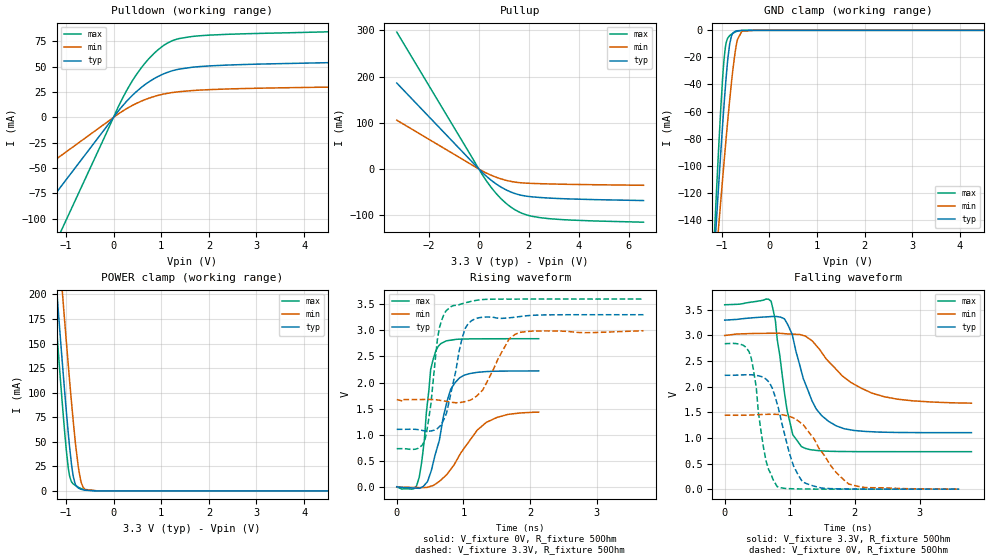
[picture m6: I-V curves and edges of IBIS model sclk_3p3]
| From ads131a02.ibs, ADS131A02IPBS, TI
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|   sclk_3p3 Model
[Model]   sclk_3p3
Model_type   I/O
Polarity   Non-Inverting
Enable   Active-Low
Vinl = 0.66
Vinh = 2.64
Vmeas = 1.65
Vref = 0
Cref = 2pF
Rref = 70
|   typ   min   max
|   (nom PVT)   (fast PVT)   (slow PVT)
C_comp   1.607e-12   1.574e-12   1.668e-12
| Where nom  PVT is Nominal Process, 3.3V, 27C
|   Fast PVT is Strong Process,  3.6V, -40C
|   Slow PVT is Weak Process,   3V, 125C
[Voltage Range]   3.3   3   3.6
|Junction Temperature
[Temperature Range]   27   125   -40
[Pullup Reference]   3.3   3   3.6
[Pulldown Reference]   0   0   0
[Power Clamp Reference]   3.3   3   3.6
[GND Clamp Reference]   0   0   0
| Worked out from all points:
|   slope of the pulldown table from 0 to 0.495 V, typ, clamps not added: 19.1 ohm
|   slope of the pullup table from 0 to 0.495 V, typ, clamps not added: 20.5 ohm
|   GND clamp passes 1 mA (typ) near -0.73 V on its own axis
|   POWER clamp passes 1 mA (typ) near -0.63 V on its own axis
|   falling waveform, V_fixture 3.3V, R_fixture 50Ohm: 20-80 % time 356ps typ, 695ps min, 204ps max; typ from 3.3 V to 1.1 V
|   rising waveform, V_fixture 0V, R_fixture 50Ohm: 20-80 % time 244ps typ, 480ps min, 130ps max; typ from 0 V to 2.22 V
|   rising waveform, V_fixture 3.3V, R_fixture 50Ohm: 20-80 % time 213ps typ, 317ps min, 156ps max; typ from 1.1 V to 3.3 V
|   falling waveform, V_fixture 0V, R_fixture 50Ohm: 20-80 % time 280ps typ, 476ps min, 184ps max; typ from 2.22 V to 0 V
[Pulldown]
|   Voltage   I(typ)   I(min)   I(max)
-3.3V     -203.7mA   -112.7mA   -335.5mA
-153.6mV  -9.48mA    -5.244mA   -15.61mA
153mV     9.485mA    5.137mA    15.86mA
462mV     24.81mA    13.45mA    41.17mA
656.7mV   32.33mA    17.49mA    53.5mA
858mV     38.51mA    20.75mA    63.65mA
1.038V    42.77mA    22.92mA    70.67mA
1.214V    45.82mA    24.42mA    75.43mA
1.647V    49.49mA    26.48mA    79.92mA
2.042V    50.92mA    27.47mA    81.33mA
5.441V    54.93mA    30.54mA    85.61mA
6.6V      57.39mA    32.04mA    89.3mA
[GND Clamp]
|   Voltage   I(typ)   I(min)   I(max)
-3.3V     -1.489A    -1.173A    -1.877A
-1.197V   -188.2mA   -201mA     -180.7mA
-1.115V   -140.9mA   -165.1mA   -120mA
-1.076V   -118.9mA   -148.3mA   -92.5mA
-985.2mV  -70.27mA   -110.1mA   -35.72mA
-924mV    -40.72mA   -85.13mA   -11.88mA
-838.2mV  -10.5mA    -52.28mA   -3.986mA
-720mV    -732.9uA   -15.72mA   -1.234mA
-672mV    -304.1uA   -6.767mA   -613.8uA
-582mV    -52.5uA    -738.4uA   -104.3uA
-330mV    -89.41nA   -746.6nA   -56.53nA
6.6V      0A         0A         0A
[Pullup]
|   Voltage   I(typ)   I(min)   I(max)
-3.3V     186.2mA    105.9mA    296.5mA
163.2mV   -8.864mA   -4.883mA   -14.59mA
462mV     -22.94mA   -12.6mA    -37.71mA
660mV     -30.98mA   -16.95mA   -50.94mA
1.15V     -46.47mA   -25.05mA   -76.84mA
1.449V    -52.89mA   -28.12mA   -88.08mA
1.734V    -56.95mA   -29.79mA   -95.74mA
2.042V    -59.45mA   -30.7mA    -101mA
2.436V    -61.34mA   -31.46mA   -104.9mA
3.633V    -64.5mA    -32.95mA   -110.1mA
6.6V      -67.97mA   -34.95mA   -114.8mA
[POWER Clamp]
|   Voltage   I(typ)   I(min)   I(max)
-3.3V     1.672A     1.701A     1.679A
-1.274V   254.9mA    325.9mA    215.1mA
-1.151V   175.7mA    247.9mA    134mA
-1.086V   135.4mA    207.7mA    93.34mA
-992.4mV  80.05mA    151.1mA    40.59mA
-920.4mV  42.32mA    109.5mA    14.15mA
-861mV    18.45mA    77.22mA    7.689mA
-808.5mV  7.107mA    51.21mA    5.653mA
-693mV    1.863mA    10.79mA    2.546mA
-597mV    682.7uA    1.477mA    880.6uA
-330mV    2.194uA    7.268uA    1.05uA
6.6V      0A         0A         0A
[Ramp]
R_load = 50
|   typ   min   max
dV/dt_r   1.33394/2.37672e-10   0.866039/4.6103e-10   1.704/1.39601e-10
dV/dt_f   1.31861/3.50263e-10   0.796462/6.51046e-10   1.72116/1.87245e-10
[Falling Waveform]
V_fixture = 3.3V
V_fixture_min = 3V
V_fixture_max = 3.6V
R_fixture = 50Ohm
|   Time   V(typ)   V(min)   V(max)
0s        3.3V       3V         3.6V
714.7ps   3.37V      3.043V     3.667V
781.2ps   3.371V     3.043V     3.283V
959.2ps   3.238V     3.031V     1.544V
1.048ns   2.971V     3.025V     1.062V
1.182ns   2.293V     3.01V      830.4mV
1.411ns   1.562V     2.801V     756.4mV
1.719ns   1.234V     2.334V     736.7mV
2.451ns   1.112V     1.806V     732mV
3.797ns   1.103V     1.679V     731.4mV
[Rising Waveform]
V_fixture = 0V
V_fixture_min = 0V
V_fixture_max = 0V
R_fixture = 50Ohm
|   Time   V(typ)   V(min)   V(max)
0s        750.8pV    33.66nV    199.1pV
256.4ps   -23.53mV   -11.57mV   -37.4mV
337.3ps   -29.58mV   -16.02mV   182.6mV
414.7ps   31.97mV    -13.22mV   909.5mV
508.2ps   273.1mV    9.834mV    2.247V
659.2ps   1.044V     126.5mV    2.744V
809.7ps   1.871V     335.4mV    2.811V
942.4ps   2.089V     607.7mV    2.831V
1.342ns   2.209V     1.234V     2.839V
2.13ns    2.222V     1.432V     2.84V
[Rising Waveform]
V_fixture = 3.3V
V_fixture_min = 3V
V_fixture_max = 3.6V
R_fixture = 50Ohm
|   Time   V(typ)   V(min)   V(max)
0s        1.102V     1.673V     731.4mV
419.5ps   1.072V     1.674V     882.6mV
512.4ps   1.071V     1.674V     1.586V
639.4ps   1.154V     1.66V      3.049V
818.6ps   1.831V     1.622V     3.459V
1.029ns   3.042V     1.636V     3.528V
1.178ns   3.223V     1.722V     3.572V
1.686ns   3.241V     2.834V     3.599V
1.847ns   3.265V     2.961V     3.6V
3.703ns   3.3V       2.993V     3.6V
[Falling Waveform]
V_fixture = 0V
V_fixture_min = 0V
V_fixture_max = 0V
R_fixture = 50Ohm
|   Time   V(typ)   V(min)   V(max)
0s        2.223V     1.443V     2.84V
374.2ps   2.234V     1.445V     2.685V
486.2ps   2.222V     1.452V     1.981V
518.6ps   2.213V     1.454V     1.499V
637.3ps   2.147V     1.461V     547mV
808.2ps   1.664V     1.46V      49.51mV
994.9ps   704.8mV    1.419V     9.975mV
1.198ns   142.2mV    1.268V     3.316mV
1.907ns   3.299mV    101.5mV    300.1uV
3.609ns   250.4uV    1.418mV    -148.9uV
